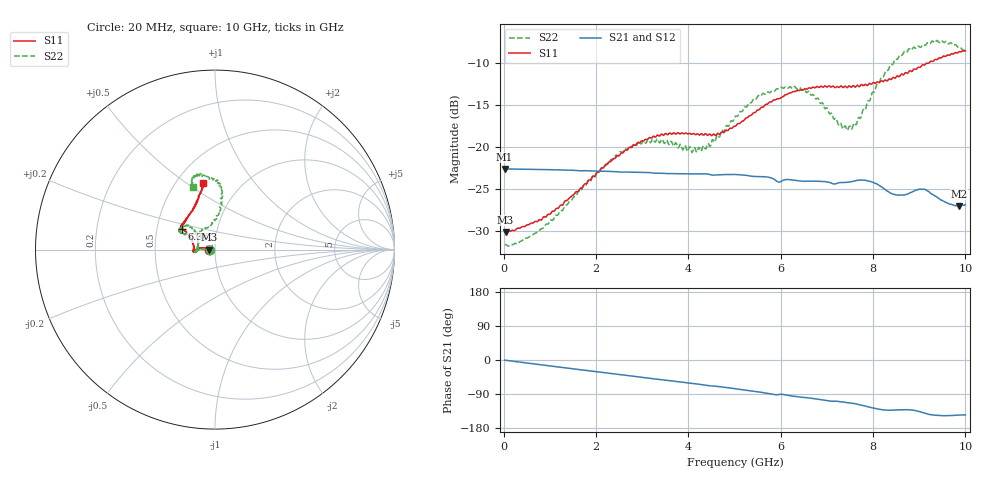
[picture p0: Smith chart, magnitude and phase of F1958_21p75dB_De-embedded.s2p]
! Integrated Device Technology
! Corporate Headquarters
! 6024 Silver Creek Valley Road
! San Jose, CA 95138  USA
! Phone:  1-408-284-8200
! Toll Free:  1-800-223-1366
! Webpage:  http://www.idt.com/
! Timing and RF Division
! 515 Groton Road, Suite 102
! Westford, MA 01886-6024
! Device:  F1958
! Description: 7-bit 0.25 dB Digital Step Attenuator
! Frequency:  0.001 -  6.000 GHz
! Package:  4x4 mm Thin QFN Plastic Package: 24 pin
! Ports:  2 RF, 12 DC
!  Pin  1  = D0
!  Pin  2  = VDD
!  Pin  3  = VMODE
!  Pin  4  = GND
!  Pin  5  = RF1  =  Port 1
!  Pin  6  = GND
!  Pin  7  = GND
!  Pin  8  = GND
!  Pin  9  = GND
!  Pin 10  = GND
!  Pin 11  = GND
!  Pin 12  = GND
!  Pin 13  = GND
!  Pin 14  = RF2  =  Port 2
!  Pin 15  = GND
!  Pin 16  = LE
!  Pin 17  = CLK
!  Pin 18  = DATA
!  Pin 19  = D6
!  Pin 20  = D5
!  Pin 21  = D4
!  Pin 22  = D3
!  Pin 23  = D2
!  Pin 24  = D1
! State:  87
! Atten State:  21.75 dB
! Voltage:  +3.30 Volts
! Current:  0.258 mA
! Data:  The device was measured on a F1958 evaluation board which has
!  individual transmission lines to the RF pins.  Data was collected
!  using a calibrated network analyzer.  The evaluation board was
!  de-embedded using Automatic Fixture Removal (AFR).
!  The reference plane is the edge of the package pin.
! Misc:
!  Action Tracker AT0419
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# GHz S dB R 50
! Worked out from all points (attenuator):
!   500 points, 20 MHz to 10 GHz, reference 50 ohm
!   highest |S21| = -22.58 dB at 20 MHz (marker M1); lowest = -27.0 dB at 9.86 GHz (marker M2)
!   lowest |S11| = -30.1 dB at 40 MHz (marker M3), VSWR 1.06, Z = 47 - j0.041 ohm
!   |S11| at or under -10 dB: start of sweep to 9.154 GHz
!   |S22| runs from -31.8 to -7.3 dB; largest |S21 - S12| = 0.00032
!   S11 on the Smith chart (normalised r, x): 20 MHz: 0.94, -0.00; 6.36 GHz: 0.67, +0.16; 10 GHz: 0.67, +0.58
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0.02  -30.09 -179.0  -22.58 -0.4  -22.58 -0.4  -31.63 -178.5
0.04  -30.12 -179.2  -22.58 -0.6  -22.58 -0.6  -31.59 -177.8
0.84  -28.52 170.8  -22.66 -13.1  -22.66 -13.1  -29.69 178.1
1.7  -24.84 170.8  -22.80 -26.1  -22.79 -26.1  -24.89 176.5
2.6  -20.59 176.7  -22.95 -39.6  -22.94 -39.7  -20.38 -179.0
3.36  -18.64 -175.8  -23.11 -51.2  -23.10 -51.3  -19.33 -171.3
4.24  -18.56 -179.1  -23.18 -64.1  -23.19 -64.2  -20.06 166.5
4.64  -18.33 171.7  -23.29 -69.9  -23.31 -69.9  -18.58 148.4
5.02  -17.50 160.7  -23.25 -76.0  -23.26 -76.0  -16.28 138.0
5.58  -15.24 150.5  -23.51 -85.2  -23.53 -85.3  -13.83 138.4
6.36  -13.23 148.1  -23.98 -96.9  -24.00 -96.8  -13.09 151.8
6.68  -12.89 146.7  -24.05 -101.3  -24.07 -101.2  -13.77 152.9
7.3  -12.70 141.0  -24.22 -110.2  -24.22 -110.2  -17.13 132.0
7.5  -12.72 138.4  -24.14 -113.3  -24.15 -113.1  -17.48 113.7
7.68  -12.69 135.5  -23.93 -117.1  -23.93 -117.0  -16.48 96.7
7.9  -12.50 129.2  -24.01 -123.7  -24.00 -123.7  -14.44 87.6
8.34  -11.88 119.3  -25.33 -132.5  -25.33 -132.6  -10.68 82.0
8.7  -11.10 112.7  -25.66 -131.0  -25.65 -131.0  -8.61 87.7
9.04  -10.37 107.2  -25.00 -137.4  -25.01 -137.3  -8.06 94.4
9.26  -9.73 105.1  -25.54 -144.5  -25.54 -144.6  -7.46 99.4
9.86  -8.64 100.1  -26.99 -145.5  -27.00 -145.2  -8.12 108.4
10  -8.50 100.1  -26.84 -144.9  -26.90 -145.0  -8.63 109.2
